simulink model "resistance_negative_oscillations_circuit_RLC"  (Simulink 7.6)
settings: Solver=ode15s  StartTime=0.0  StopTime=12  RelTol=1e-3
InitFcn:
  | R=1; L=0.01; C=1e-3;
StopFcn:
  | close all
  | load mesures_IL_UC.mat
  | plot(x(1,:),x(2,:),x(1,:),x(3,:) )
  | grid
  | title('Tension aux bornes de C et courant dans l''inductance')
  | xlabel('temps')
libraries: powerlib x13, powerlib_extras x1

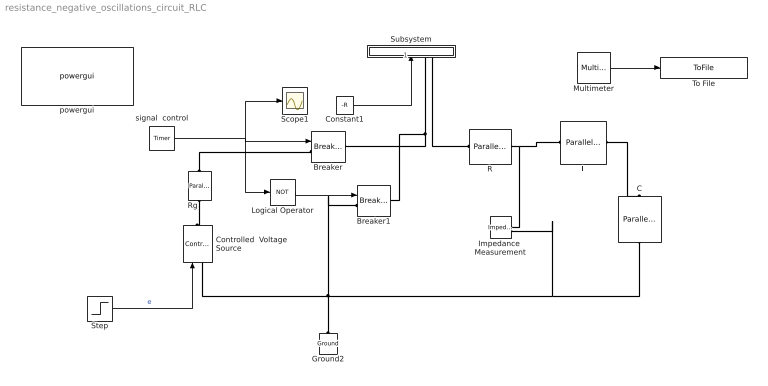
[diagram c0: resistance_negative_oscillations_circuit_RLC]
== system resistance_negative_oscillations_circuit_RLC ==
  Breaker : powerlib/Elements/Breaker  DialogController=POWERSYS.PowerSysDialog  SystemSampleTime=-1  BreakerResistance=1e-4  InitialState=1  SnubberResistance=1e6  SnubberCapacitance=inf  SwitchingTimes="[ 4/60  5/60 ]"  External=on  Measurements=Branch current  MoreParameters=off  NoBreakLoop=off
  Breaker1 : powerlib/Elements/Breaker  DialogController=POWERSYS.PowerSysDialog  SystemSampleTime=-1  BreakerResistance=1e-4  InitialState=0  SnubberResistance=1e6  SnubberCapacitance=inf  SwitchingTimes="[ 4/60  5/60 ]"  External=on  Measurements=Branch current  MoreParameters=off  NoBreakLoop=off
  C : powerlib/Elements/Parallel RLC Branch  DialogController=POWERSYS.PowerSysDialog  PhysicalDomain=powersysdomain  SubClassName=unknown  LeftPortType=p1  RightPortType=p1  LConnTagsString=a  RConnTagsString=__new0  BranchType=C  Resistance=1  Inductance=1e-3  SetiL0=off  InitialCurrent=0  Capacitance=C  Setx0=on  InitialVoltage=0.5  Measurements=Branch voltage
  Constant1 : Constant  Value=-R
  Controlled  Voltage Source : powerlib/Electrical Sources/Controlled Voltage Source  DialogController=POWERSYS.PowerSysDialog  SystemSampleTime=-1  Initialize=on  Source_Type=AC  Amplitude=0  Phase=0  Frequency=0  Measurements=None
  Ground2 : powerlib/Elements/Ground  DialogController=POWERSYS.PowerSysDialog  PhysicalDomain=powersysdomain  SubClassName=unknown  LeftPortType=p1  RightPortType=p1  LConnTagsString=a
  Impedance  Measurement : powerlib/Measurements/Impedance Measurement  DialogController=POWERSYS.PowerSysDialog  PhysicalDomain=powersysdomain  SubClassName=unknown  LeftPortType=p1  RightPortType=p1  LConnTagsString=+|-  Factor=1
  L : powerlib/Elements/Parallel RLC Branch  DialogController=POWERSYS.PowerSysDialog  PhysicalDomain=powersysdomain  SubClassName=unknown  LeftPortType=p1  RightPortType=p1  LConnTagsString=a  RConnTagsString=__new0  BranchType=L  Resistance=1  Inductance=L  SetiL0=on  InitialCurrent=1  Capacitance=1e-6  Setx0=off  InitialVoltage=0  Measurements=Branch current
  Logical Operator : Logic  Operator=NOT  AllPortsSameDT=off  OutDataTypeStr=boolean
  Multimeter : powerlib/Measurements/Multimeter  SystemSampleTime=-1  PhasorSimulation=off  OutputType=Complex  sel=[1 2]  L=4  Gain=[1 1]  yselected={'Ub: C','Ib: L'};  PSBOutputType=1  PSBequivalent=0  AxesSetting=[0,0.1,-100,100]  Display=0  SavedBlockNames=-11
  R : powerlib/Elements/Parallel RLC Branch  DialogController=POWERSYS.PowerSysDialog  PhysicalDomain=powersysdomain  SubClassName=unknown  LeftPortType=p1  RightPortType=p1  LConnTagsString=a  RConnTagsString=__new0  BranchType=R  Resistance=R  Inductance=10e-03  SetiL0=off  InitialCurrent=0  Capacitance=[]  Setx0=off  InitialVoltage=0  Measurements=None
  Rg : powerlib/Elements/Parallel RLC Branch  DialogController=POWERSYS.PowerSysDialog  PhysicalDomain=powersysdomain  SubClassName=unknown  LeftPortType=p1  RightPortType=p1  LConnTagsString=a  RConnTagsString=__new0  BranchType=R  Resistance=1e-9  Inductance=10e-03  SetiL0=off  InitialCurrent=0  Capacitance=[]  Setx0=off  InitialVoltage=0  Measurements=None
  Scope1 : Scope
  Step : Step  Time=0  SampleTime=0
  Subsystem : Subsystem
  To File : ToFile  Filename=mesures_IL_UC  MatrixName=x
  powergui : powerlib/powergui  SystemSampleTime=-1  SimulationMode=Continuous  SampleTime=0  frequency=60  SPID=on  DisableSnubberDevices=on  DisableRonSwitches=on  DisableVfSwitches=on  SwTol=0  Interpol=off  frequencyindice=0  echomessages=off  HookPort=off  DisplayEquations=off  FunctionMessages=off  EnableUseOfTLC=off  x0status=zero  RestoreLinks=warning  ResistiveCurrentMeasurement=off  Frange=[1:2:1000]  Ylog=off  Xlog=on  ShowGrid=on  save=off  variable=ZData  ZoomFFT=on  StartTime=0.0  cycles=1  DisplayStyle=1  fundamental=60  FreqAxis=off  MaxFrequency=1000  frequencyindicesteady=60  RmsSteady=1  display=off  Ts=0  methode=off
  signal  control : powerlib_extras/Control  Blocks/Timer  DialogController=POWERSYS.PowerSysDialog  SystemSampleTime=-1  t=[0 1 5 10]  e=[1 1 0 0]
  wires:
  Step/1 -> Controlled  Voltage Source/1  "e"
  signal  control/1 -> Scope1/1, Breaker/1, Logical Operator/1
  Constant1/1 -> Subsystem/1(R)
  Multimeter/1 -> To File/1
  Logical Operator/1 -> Breaker1/1
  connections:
  C/RConn1 -- Controlled  Voltage Source/LConn1 -- Ground2/LConn1 -- Breaker1/LConn1 -- Impedance  Measurement/LConn2
  R/RConn1 -- L/LConn1 -- Impedance  Measurement/LConn1
  Subsystem/LConn1 -- Breaker/RConn1 -- Breaker1/RConn1
  Subsystem/LConn2 -- R/LConn1
  L/RConn1 -- C/LConn1
  Rg/RConn1 -- Controlled  Voltage Source/RConn1
  Rg/LConn1 -- Breaker/LConn1

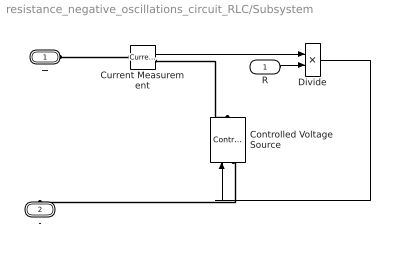
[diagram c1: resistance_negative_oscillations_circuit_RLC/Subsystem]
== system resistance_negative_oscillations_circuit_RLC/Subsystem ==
  R : Inport
  Controlled Voltage Source : powerlib/Electrical Sources/Controlled Voltage Source  DialogController=POWERSYS.PowerSysDialog  SystemSampleTime=-1  Initialize=on  Source_Type=AC  Amplitude=0  Phase=0  Frequency=60  Measurements=None
  Current Measurement : powerlib/Measurements/Current Measurement  DialogController=POWERSYS.PowerSysDialog  SystemSampleTime=-1  PhasorSimulation=off  OutputType=Complex  PSBequivalent=0
  Divide : Product  Inputs=**
  + : PMIOPort  Port=1  Side=Left
  - : PMIOPort  Port=2  Side=Left
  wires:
  R/1 -> Divide/2
  Divide/1 -> Controlled Voltage Source/1
  Current Measurement/1 -> Divide/1
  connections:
  -/RConn1 -- Controlled Voltage Source/LConn1
  +/RConn1 -- Current Measurement/LConn1
  Current Measurement/RConn1 -- Controlled Voltage Source/RConn1
